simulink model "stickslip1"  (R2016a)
settings: Solver=ode45  SolverMode=SingleTasking  StartTime=0.0  StopTime=10  FixedStep=0.001  MaxStep=0.01  RelTol=1e-3  AbsTol=1e-6
InitFcn:
  | m = 1;
undefined symbols (not defined in the file or in its folder): FN, mug, muh

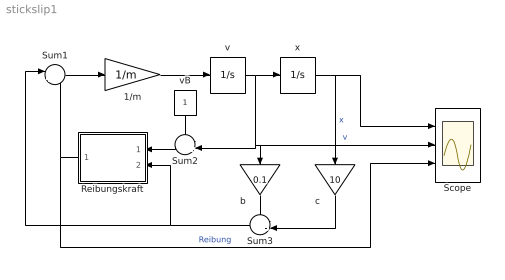
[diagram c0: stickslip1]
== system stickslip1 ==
  note: .
  1/m : Gain  Gain=1/m
  Reibungskraft : Subsystem
  Scope : Scope  NumInputPorts=3
  Sum1 : Sum  Inputs=|++
  Sum2 : Sum  Inputs=-+|
  Sum3 : Sum  Inputs=--|
  b : Gain  Gain=0.1
  c : Gain  Gain=10
  v : Integrator
  vB : Constant
  x : Integrator  UpperSaturationLimit=100  LowerSaturationLimit=-100
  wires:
  x/1 -> Scope/1, c/1  "x"
  Sum1/1 -> 1/m/1
  v/1 -> x/1, Sum2/2, b/1, Scope/2  "v"
  1/m/1 -> v/1
  Reibungskraft/1(FR) -> Scope/3, Sum1/2  "Reibung"
  Sum3/1 -> Sum1/1, Reibungskraft/2(Fext)
  Sum2/1 -> Reibungskraft/1(v)
  vB/1 -> Sum2/1
  b/1 -> Sum3/1
  c/1 -> Sum3/2

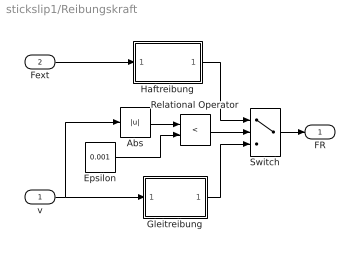
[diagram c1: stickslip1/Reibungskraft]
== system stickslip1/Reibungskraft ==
  v : Inport
  Fext : Inport  Port=2
  Abs : Abs
  Epsilon : Constant  Value=0.001
  Gleitreibung : Subsystem
  Haftreibung : Subsystem
  Relational Operator : RelationalOperator  Operator=<
  Switch : Switch  Threshold=0.5
  FR : Outport
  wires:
  Switch/1 -> FR/1
  Fext/1 -> Haftreibung/1(Fext)
  v/1 -> Gleitreibung/1(v), Abs/1
  Abs/1 -> Relational Operator/1
  Epsilon/1 -> Relational Operator/2
  Haftreibung/1(Fh) -> Switch/1
  Gleitreibung/1(Fg) -> Switch/3
  Relational Operator/1 -> Switch/2

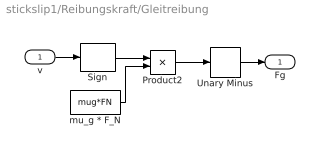
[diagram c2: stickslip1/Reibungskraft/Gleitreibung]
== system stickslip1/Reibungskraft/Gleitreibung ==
  v : Inport
  Product2 : Product
  Sign : Signum
  Unary Minus : UnaryMinus
  mu_g * F_N : Constant  Value=mug*FN
  Fg : Outport
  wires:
  mu_g * F_N/1 -> Product2/2
  Sign/1 -> Product2/1
  v/1 -> Sign/1
  Product2/1 -> Unary Minus/1
  Unary Minus/1 -> Fg/1

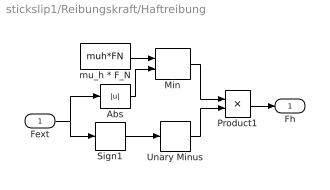
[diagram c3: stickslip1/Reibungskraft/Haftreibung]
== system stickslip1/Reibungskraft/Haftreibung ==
  Fext : Inport
  Abs : Abs
  Min : MinMax  Inputs=2
  Product1 : Product
  Sign1 : Signum
  Unary Minus : UnaryMinus
  mu_h * F_N : Constant  Value=muh*FN
  Fh : Outport
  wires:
  Abs/1 -> Min/2
  mu_h * F_N/1 -> Min/1
  Min/1 -> Product1/1
  Fext/1 -> Abs/1, Sign1/1
  Product1/1 -> Fh/1
  Sign1/1 -> Unary Minus/1
  Unary Minus/1 -> Product1/2
